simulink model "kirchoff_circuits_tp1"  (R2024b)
settings: Solver=ode23s  StartTime=0.0  StopTime=0.01  RelTol=1e-3  EnableMultiTasking=on
libraries: fl_lib x9, nesl_utility x5, spspowerguiLib x1

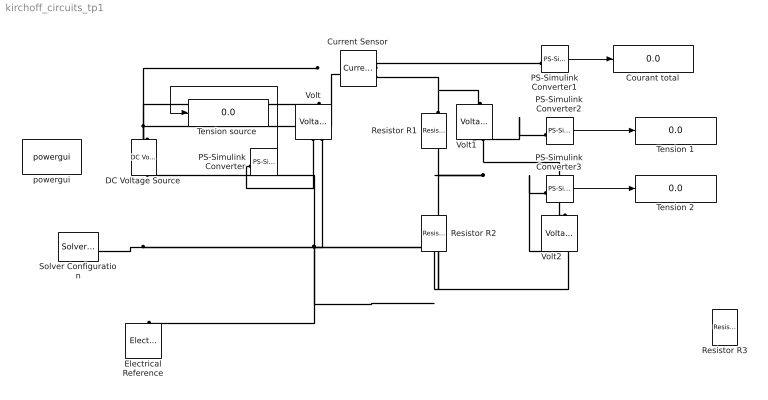
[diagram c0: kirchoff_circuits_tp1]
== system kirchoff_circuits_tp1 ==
  Courant total : Display
  Current Sensor : fl_lib/Electrical/Electrical Sensors/Current Sensor
  DC Voltage Source : fl_lib/Electrical/Electrical Sources/DC Voltage Source  v0=5 V
  Electrical Reference : fl_lib/Electrical/Electrical Elements/Electrical Reference
  PS-Simulink Converter : nesl_utility/PS-Simulink Converter  PhysicalDomain=network_engine_domain  SubClassName=ps_output  LeftPortType=input  RightPortType=output  PseudoPeriodic=off  Frequencies=[]  VectorFormat=1-D array  Unit=V  AffineConversion=off
  PS-Simulink Converter1 : nesl_utility/PS-Simulink Converter  PhysicalDomain=network_engine_domain  SubClassName=ps_output  LeftPortType=input  RightPortType=output  PseudoPeriodic=off  Frequencies=[]  VectorFormat=1-D array  Unit=A  AffineConversion=off
  PS-Simulink Converter2 : nesl_utility/PS-Simulink Converter  PhysicalDomain=network_engine_domain  SubClassName=ps_output  LeftPortType=input  RightPortType=output  PseudoPeriodic=off  Frequencies=[]  VectorFormat=1-D array  Unit=V  AffineConversion=off
  PS-Simulink Converter3 : nesl_utility/PS-Simulink Converter  PhysicalDomain=network_engine_domain  SubClassName=ps_output  LeftPortType=input  RightPortType=output  PseudoPeriodic=off  Frequencies=[]  VectorFormat=1-D array  Unit=V  AffineConversion=off
  Resistor R1 : fl_lib/Electrical/Electrical Elements/Resistor  R=100 Ohm  i_specify=off  i_priority=None  i=0 A  i_nominal_specify=off  i_nominal_value=1  i_nominal_unit=A  v_specify=off  v_priority=None  v=0 V  v_nominal_specify=off  v_nominal_value=1  v_nominal_unit=V
  Resistor R2 : fl_lib/Electrical/Electrical Elements/Resistor  R=0 Ohm  i_specify=off  i_priority=None  i=0 A  i_nominal_specify=off  i_nominal_value=1  i_nominal_unit=A  v_specify=off  v_priority=None  v=0 V  v_nominal_specify=off  v_nominal_value=1  v_nominal_unit=V
  Resistor R3 : fl_lib/Electrical/Electrical Elements/Resistor  R=220 Ohm  i_specify=off  i_priority=None  i=0 A  i_nominal_specify=off  i_nominal_value=1  i_nominal_unit=A  v_specify=off  v_priority=None  v=0 V  v_nominal_specify=off  v_nominal_value=1  v_nominal_unit=V
  Solver Configuration : nesl_utility/Solver Configuration  PhysicalDomain=network_engine_domain  SubClassName=solver  LeftPortType=input  RightPortType=generic  Tones=[]  Harmonics=[]  SimulateNoise=off  Profile=off  UseLocalSampling=off  EnableSwitchedLinearOptims=on  FrequencyDomain=off  UseCCode=off  RelTol=0.001  AbsTol=1e-06  MinStep=1e-09  ToWorkspace=off  RevertToSquareIcSolve=off  NumHomotopyIterations=100  PhasorMode=off  PhasorModeNumHarmonics=1  ConsistencySolver=NEWTON_FTOL  IndexReductionMethod=DerivativeReplacement  DoDC=off  ResidualTolerance=1e-9  ConsistencyTolSource=GLOBAL  ConsistencyAbsTol=0.001  ConsistencyRelTol=0.001  ConsistencyTolFactor=0.001  UseLocalSolver=off  LocalSolverChoice=NE_BACKWARD_EULER_ADVANCER  ResolveIndetEquations=on  FunctionEvalNumThread=1  LocalSolverSampleTime=.001  DoFixedCost=off  MaxNonlinIter=3  MaxModeIter=2  ComputeImpulses=off  ImpulseIterations=2  LinearAlgebra=Sparse  LinearAlgebraNumThread=0  EquationFormulation=NE_TIME_EF  DelaysMemoryBudget=1024  AutomaticFiltering=on  FilteringTimeConstant=0.001  PartitionStorageMethod=AS_NEEDED  PartitionMemoryBudget=1024  PartitionMethod=FAST  MultibodyUseLocalSolver=off  MultibodyLocalSolverChoice=ODE1  MultibodyLocalSolverSampleTime=0.001
  Tension 1 : Display
  Tension 2 : Display
  "Tension source " : Display
  Volt : fl_lib/Electrical/Electrical Sensors/Voltage Sensor
  Volt1 : fl_lib/Electrical/Electrical Sensors/Voltage Sensor
  Volt2 : fl_lib/Electrical/Electrical Sensors/Voltage Sensor
  powergui : spspowerguiLib/powergui  Priority=1  SimulationMode=Continuous  SampleTime=50e-6  frequency=60  Iterations=50  frequencyindice=17  Pbase=100e6  ErrMax=1e-4  UnitsV=V  UnitsW=W  buscounter=0  FunctionMessages=off  echomessages=off  EnableUseOfTLC=off  CurrentSourceSwitches=on  DisableSnubberDevices=off  DisableRonSwitches=off  DisableVfSwitches=off  DisplayEquations=off  AutomaticDiscreteSolvers=off  SolverType=Tustin  Interpol=off  ExternalGateDelay=off  methode=off  Ts=100  x0status=blocks  SPID=off  SwTol=0  HookPort=off  NonlinearTolerance=1e-4  nMaxIteration=100  ContinueOnMaxIteration=off  RestoreLinks=warning  ResistiveCurrentMeasurement=off  Frange=[0:2:500]  Ylog=off  Xlog=on  ShowGrid=off  save=off  variable=ZData  structure=0  ZoomFFT=off  StartTime=0.0  cycles=1  DisplayStyle=1  fundamental=60  FreqAxis=off  MaxFrequency=1000  frequencyindicesteady=1  RmsSteady=1  display=off
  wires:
  PS-Simulink Converter1/1 -> Courant total/1
  PS-Simulink Converter/1 -> "Tension source "/1
  PS-Simulink Converter2/1 -> Tension 1/1
  PS-Simulink Converter3/1 -> Tension 2/1
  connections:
  Solver Configuration/RConn1 -- Electrical Reference/LConn1 -- DC Voltage Source/RConn1 -- Resistor R2/RConn1 -- Volt2/RConn2 -- Volt/RConn2
  DC Voltage Source/LConn1 -- Volt/LConn1 -- Current Sensor/LConn1
  Current Sensor/RConn1 -- PS-Simulink Converter1/LConn1
  Resistor R1/LConn1 -- Current Sensor/RConn2 -- Volt1/LConn1
  Volt/RConn1 -- PS-Simulink Converter/LConn1
  Volt1/RConn1 -- PS-Simulink Converter2/LConn1
  Volt2/RConn1 -- PS-Simulink Converter3/LConn1
  Volt1/RConn2 -- Resistor R2/LConn1 -- Resistor R1/RConn1 -- Volt2/LConn1
